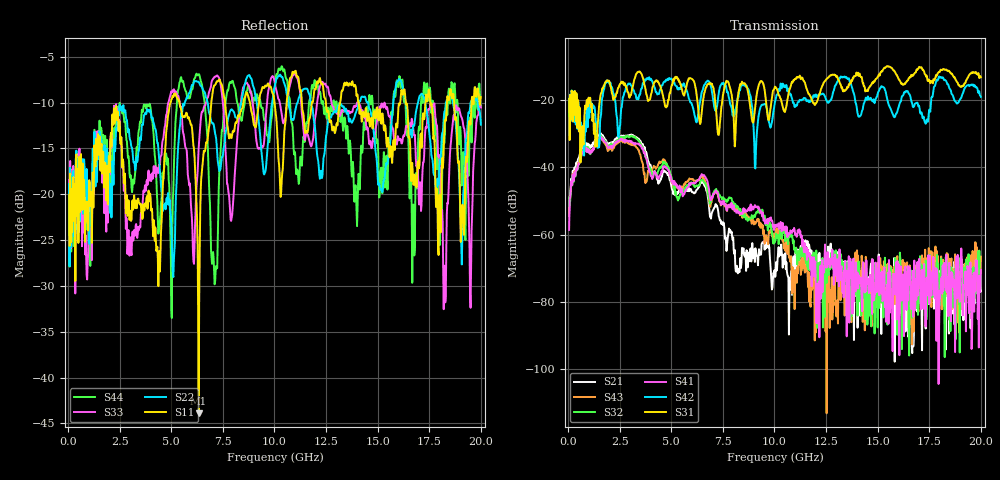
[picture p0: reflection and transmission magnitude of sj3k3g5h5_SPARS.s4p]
! FILE: E:\users\goganessyan\GBX_Backplane\FR408_backplane\1m_INBOUND_FEXT\sj3k3g5h5_SPARS.s4p
# MHZ S RI R 50.00
! FREQ  S11  S12  S13  S14
!  S21  S22  S23  S24
!  S31  S32  S33  S34
!  S41  S42  S43  S44
!  REAL  IMAG  REAL  IMAG  REAL  IMAG  REAL  IMAG
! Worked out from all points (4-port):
!   799 points, 50 MHz to 20 GHz, reference 50 ohm
!   strongest paths, dB at 50 MHz, 5.025 GHz, 10.03 GHz, 15.03 GHz, 20 GHz:
!     S31: -19.8, -15.6, -16.1, -13.1, -13.3
!     S42: -19.7, -14.0, -20.7, -17.7, -19.1
!     S41: -58.6, -44.4, -57.1, -74.0, -70.4
!     S32: -51.6, -43.2, -61.9, -72.3, -72.2
!     S43: -53.7, -44.6, -60.1, -74.8, -66.5
!     S21: -54.4, -46.3, -72.6, -75.1, -76.8
!   lowest |S11| = -43.9 dB at 6.325 GHz (marker M1), VSWR 1.01, Z = 49.7 + j0.542 ohm
!   |S11| at or under -10 dB: start of sweep to 4.968 GHz; 5.392 GHz to 6.94 GHz (1.548 GHz wide, 25.1 % of centre); 14.08 GHz to 16.09 GHz (2.014 GHz wide, 13.4 % of centre)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
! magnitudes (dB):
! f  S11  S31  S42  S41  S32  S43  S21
! 50 MHz  -20.1  -19.8  -19.7  -58.6  -51.6  -53.7  -54.4
! 1.55 GHz  -15.4  -19.7  -26.4  -31.3  -31.1  -31.4  -30.3
! 6.325 GHz  -43.9  -24.3  -23.4  -43.7  -45.3  -43.8  -46.0
! 7.15 GHz  -8.0  -21.9  -23.2  -47.1  -46.8  -47.6  -50.9
! 11.75 GHz  -11.2  -19.0  -20.6  -70.2  -67.3  -81.4  -65.4
! 18.25 GHz  -12.0  -11.1  -14.1  -71.3  -96.3  -76.7  -72.9
! 20 GHz  -9.4  -13.3  -19.1  -70.4  -72.2  -66.5  -76.8
